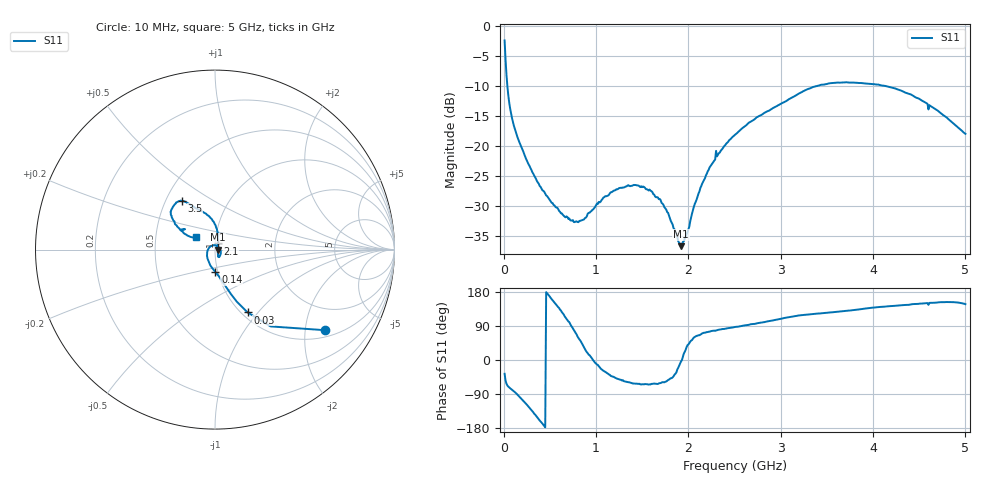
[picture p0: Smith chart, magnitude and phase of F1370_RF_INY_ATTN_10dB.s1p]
! S-parameters for RF_INY input IDT F1370 DPD Demodulator
! Date Measured:  2015-11-25  RGG
!  Port 1 = Pin 3 = RF_INY
! STATE: RF_INY selected, 10 dB attenuation (Gain = Gmax - 10 dB)
! RF Frequency:  10 MHz to 5000 MHz
! RF_INX, IF_I+, IF_I-, IF_Q+, and IF_Q- terminated
! 2300 MHz, 0 dBm signal applied to LO_IN
! Vcc = +5.00 Volts  Icc = approx 275 mA
! NOTES:  The device was measured on a custom printed circuit evaluation board with individual 50 ohm
!  microstrip lines to the RF and LO pins. The 50 ohm microstrip lines were de-embedded using reference
!  plane extensions
! Instrument Manufacturer:  Agilent Technologies
! Instrument Model:  E5071C
! Instrument Serial Number:  MY46419053
! Instrument Firmware Rev:  A.11.31
# HZ  S  RI R 50.00
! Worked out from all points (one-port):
!   500 points, 10 MHz to 5 GHz, reference 50 ohm
!   lowest |S11| = -36.7 dB at 1.92 GHz (marker M1), VSWR 1.03, Z = 51.5 - j0.106 ohm
!   |S11| at or under -10 dB: 39.82 MHz to 3.394 GHz (3.354 GHz wide, 195 % of centre); 4.135 GHz to end of sweep
!   S11 on the Smith chart (normalised r, x): 10 MHz: 1.21, -2.54; 30 MHz: 1.07, -0.88; 140 MHz: 0.97, -0.25; 2.1 GHz: 1.03, +0.07; 3.5 GHz: 0.60, +0.37; 5 GHz: 0.80, +0.11
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1e7  0.6101 -0.4488
3e7  0.1817 -0.35
4e7  0.1218 -0.2905
6e7  0.0689 -0.219
9e7  0.0344 -0.1676
1.4e8  0.00202 -0.124
3.8e8  -0.0445 -0.0194
6.4e8  -0.0147 0.0224
7.5e8  0.00295 0.024
8.5e8  0.0178 0.0163
1.08e9  0.0327 -0.0177
1.26e9  0.0276 -0.0352
1.43e9  0.0218 -0.0421
1.6e9  0.0191 -0.0375
1.76e9  0.0163 -0.0248
1.89e9  0.0151 -0.00568
1.92e9  0.0146 -0.00103
1.99e9  0.0149 0.012
2.1e9  0.0165 0.0342
2.28e9  0.0164 0.0738
2.51e9  0.0058 0.1249
3.13e9  -0.1077 0.2318
3.5e9  -0.1855 0.271
3.76e9  -0.2211 0.2544
4.13e9  -0.246 0.1998
4.38e9  -0.2257 0.1548
4.68e9  -0.1773 0.0965
5e9  -0.1063 0.0684
